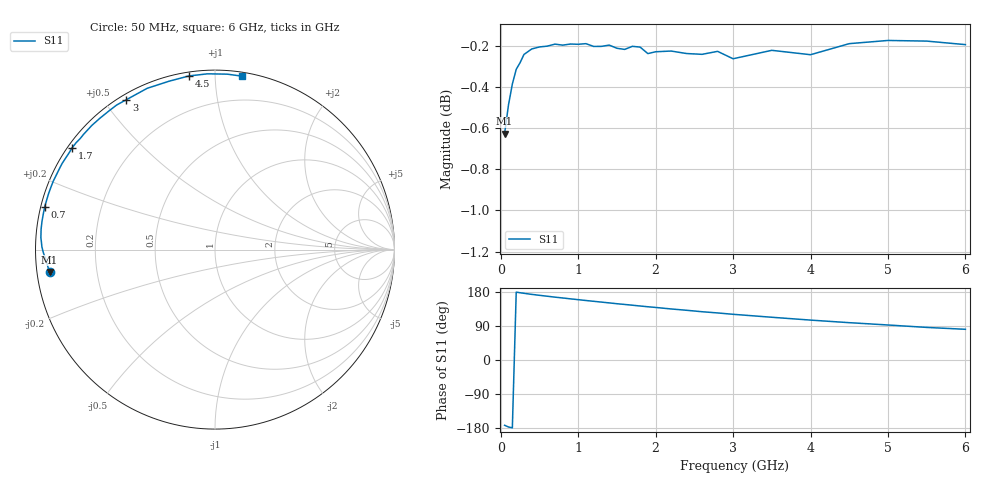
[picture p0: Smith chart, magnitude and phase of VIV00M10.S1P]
! Infineon Technologies  Discrete & RF Semiconductors
! BB 804
! Si Tuning Diode in SOT23
! VR =
! S-Parameters:  July  1999
# GHz  S  MA  R  50
!  f  S11
! GHz  MAG  ANG
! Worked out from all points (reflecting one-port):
!   34 points, 50 MHz to 6 GHz, reference 50 ohm
!   lowest |S11| = -0.6 dB at 50 MHz (marker M1), VSWR 27.75, Z = 1.81 - j3.36 ohm
!   phase of S11 starts at -172 deg and turns -107 deg over the sweep
!   S11 on the Smith chart (normalised r, x): 50 MHz: 0.04, -0.07; 700 MHz: 0.01, +0.12; 1.7 GHz: 0.01, +0.32; 3 GHz: 0.02, +0.57; 4.5 GHz: 0.02, +0.86; 6 GHz: 0.03, +1.17
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0.05  0.9304 -172.3
0.1  0.9454 -176.8
0.15  0.9566 -179.0
0.2  0.9645 179.1
0.3  0.9726 176.0
0.4  0.9756 173.2
0.5  0.9767 170.7
0.7  0.9782 165.9
0.8  0.9777 163.7
1.1  0.9785 157.0
1.4  0.9777 150.7
1.5  0.9759 148.5
1.6  0.9753 146.6
1.7  0.977 144.6
1.8  0.9766 142.5
1.9  0.973 140.5
2  0.974 138.7
2.2  0.9744 134.7
2.4  0.9731 131.2
2.6  0.9726 127.4
2.8  0.9743 124.2
3  0.9702 120.6
3.5  0.9748 112.8
4  0.9724 105.3
4.5  0.9785 98.5
5  0.9802 92.4
5.5  0.9799 86.0
6  0.9779 81.0
